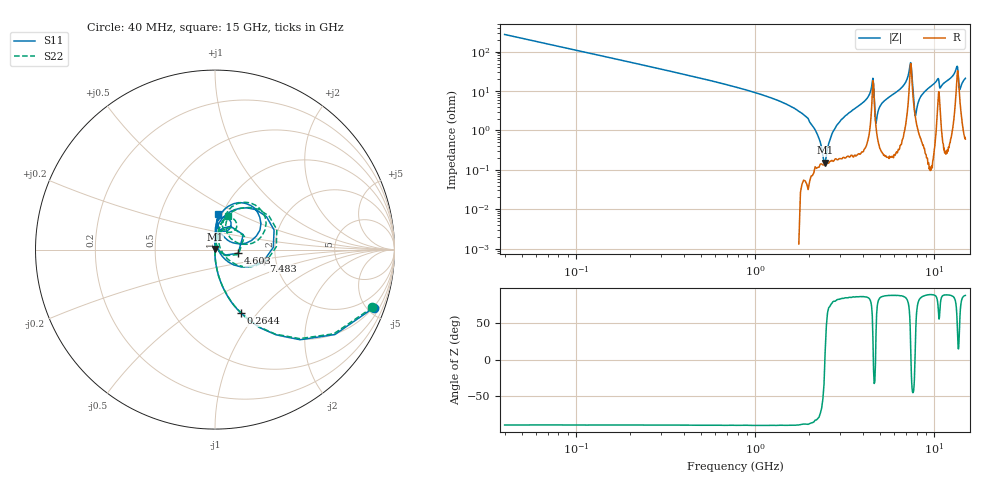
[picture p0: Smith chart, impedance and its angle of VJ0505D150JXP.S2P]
! VJ0505D150JXP
! MLCC placed on 25 mil thick microstrip substrate in series configuraton.
! DATE 06/29/2018  09:02
! CORRECTED  DATA
# GHz  S  MA  R  50.00
!  FREQ  S11M  S11A  S21M  S21A  S12M  S12A  S22M  S22A
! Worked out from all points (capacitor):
!   401 points, 40 MHz to 15 GHz, reference 50 ohm
!   read as one part in series: C = 14.6 pF near 114.8 MHz
!   lowest |Z| = 151 mohm at 2.471 GHz (marker M1)
!   series resonance near 2.462 GHz, so ESL is about 290 pH
!   S11 on the Smith chart (normalised r, x): 40 MHz: 0.95, -5.48; 264.4 MHz: 1.00, -0.82; 4.603 GHz: 1.29, -0.05; 7.483 GHz: 1.73, -0.23; 15 GHz: 0.96, +0.39
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0.04  0.9419 -20.1  0.3438 69.9  0.3444 69.9  0.9345 -20.2
0.2644  0.3797 -67.9  0.925 22.3  0.9258 22.3  0.3766 -67.8
1.91  0.02113 -91.7  0.9973 1.5  0.9986 1.5  0.02102 -89.5
2.1718  0.008474 -94.5  0.9977 0.7  0.9974 0.7  0.008133 -83.8
2.3588  0.001121 -118.5  0.9971 0.3  0.998 0.4  0.001482 -27.5
2.471  0.002917 98.3  0.9973 0.1  0.9978 0.2  0.003238 63.5
2.5458  0.005935 96.6  0.9973 -0.0  0.9977 0.0  0.006444 74.3
3.1068  0.02328 90.3  0.9965 -1.0  0.9969 -1.0  0.0237 82.5
4.528  0.156 56.0  0.9145 -7.5  0.9148 -7.4  0.1563 52.1
4.6028  0.1305 -9.1  0.8703 2.1  0.8706 2.2  0.1334 -12.1
4.7524  0.01639 56.4  0.9867 -0.3  0.9872 -0.3  0.01813 42.4
5.0516  0.04861 88.8  0.9945 -2.3  0.995 -2.3  0.04773 81.3
7.2582  0.2681 59.1  0.8825 -14.6  0.8836 -14.6  0.2762 57.0
7.4826  0.2795 -12.7  0.7211 5.4  0.7214 5.5  0.2964 -11.5
7.52  0.2247 -24.8  0.7929 7.4  0.7934 7.4  0.24 -22.7
7.8566  0.01625 23.5  0.9754 0.0  0.9763 0.1  0.03076 10.9
8.4176  0.07156 88.4  0.9897 -3.9  0.9905 -3.8  0.07432 75.4
10.0258  0.1521 86.3  0.9839 -8.6  0.9844 -8.7  0.1572 75.3
12.5316  0.2097 79.7  0.9691 -12.6  0.9691 -12.8  0.2181 71.9
13.4666  0.3159 41.6  0.7788 -16.2  0.7791 -16.3  0.3381 38.4
13.9154  0.0861 48.3  0.927 -4.6  0.9272 -4.6  0.1082 33.9
15  0.198 84.4  0.9724 -12.4  0.9727 -12.4  0.1985 68.4
